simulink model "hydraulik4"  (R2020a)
settings: Solver=ode45  StartTime=0.0  StopTime=2  MaxStep=0.01  RelTol=1e-3  EnableMultiTasking=on
InitFcn:
  | pa = 1e5;

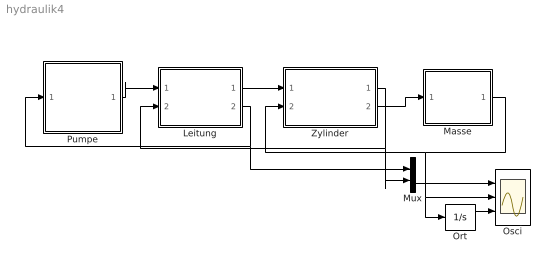
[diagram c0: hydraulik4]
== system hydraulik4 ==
  note: .
  Leitung : Subsystem  mask(Leitung (laminar)){R=8e7}
      mask prompts: R "laminarer Stroemungswiderstand"
  Masse : Subsystem  mask(Masse){m=500}
      mask prompts: m "Masse"
  Mux : Mux  Inputs=2
  Ort : Integrator
  Osci : Scope  NumInputPorts=3
  Pumpe : Subsystem  mask(Pumpe){Qzu=0.001, R=1e9}
      mask prompts: Qzu "Volumenstrom der Pumpe"; R "Stroemungswiderstand der Leckstroemung"
      mask help: Pumpe mit Leckstrom gegen Aussendruck
  Zylinder : Subsystem  mask(Zylinder){A=1e-3, V0=2.5e-5, K=1.15e9, p0=1e5}
      mask prompts: A "Kolbenflaeche"; V0 "Zylindervolumen bei x = 0"; K "Kompressionsmodul"; p0 "Anfangsdruck"
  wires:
  Pumpe/1(Q) -> Leitung/1(Q1)
  Leitung/2(p1) -> Mux/1, Pumpe/1(p)
  Leitung/1(Q2) -> Zylinder/1(Q)
  Zylinder/1(p) -> Mux/2, Leitung/2(p2)
  Zylinder/2(F) -> Masse/1(F)
  Masse/1(v) -> Ort/1, Osci/2, Zylinder/2(v)
  Mux/1 -> Osci/1
  Ort/1 -> Osci/3

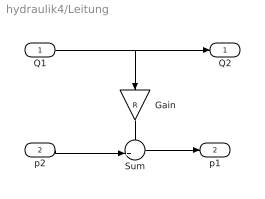
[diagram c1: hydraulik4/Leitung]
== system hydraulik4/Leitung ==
  Q1 : Inport
  p2 : Inport  Port=2
  Gain : Gain  Gain=R
  Sum : Sum  Inputs=++|
  Q2 : Outport
  p1 : Outport  Port=2
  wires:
  Q1/1 -> Q2/1, Gain/1
  p2/1 -> Sum/2
  Sum/1 -> p1/1
  Gain/1 -> Sum/1

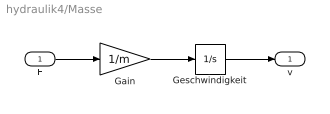
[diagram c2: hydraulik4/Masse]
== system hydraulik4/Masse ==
  F : Inport
  Gain : Gain  Gain=1/m
  Geschwindigkeit : Integrator
  v : Outport
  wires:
  F/1 -> Gain/1
  Geschwindigkeit/1 -> v/1
  Gain/1 -> Geschwindigkeit/1

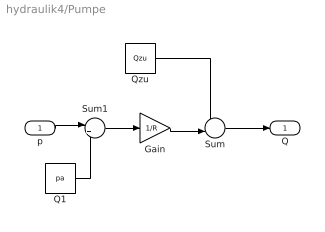
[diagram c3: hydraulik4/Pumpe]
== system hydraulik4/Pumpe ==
  p : Inport
  Gain : Gain  Gain=1/R
  Q1 : Constant  Value=pa
  Qzu : Constant  Value=Qzu
  Sum : Sum  Inputs=+-|
  Sum1 : Sum  Inputs=|+-
  Q : Outport
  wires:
  Qzu/1 -> Sum/1
  Gain/1 -> Sum/2
  Sum/1 -> Q/1
  p/1 -> Sum1/1
  Sum1/1 -> Gain/1
  Q1/1 -> Sum1/2

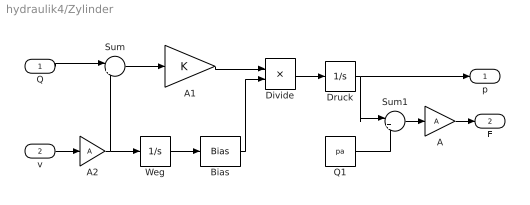
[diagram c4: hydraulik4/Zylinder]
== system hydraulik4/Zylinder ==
  Q : Inport
  v : Inport  Port=2
  A : Gain  Gain=A
  A1 : Gain  Gain=K
  A2 : Gain  Gain=A
  Bias : Bias  Bias=V0
  Divide : Product  Inputs=*/
  Druck : Integrator  InitialCondition=p0  LimitOutput=on  LowerSaturationLimit=0
  Q1 : Constant  Value=pa
  Sum : Sum  Inputs=|+-
  Sum1 : Sum  Inputs=|+-
  Weg : Integrator
  p : Outport
  F : Outport  Port=2
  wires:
  A/1 -> F/1
  Druck/1 -> p/1, Sum1/1
  v/1 -> A2/1
  Weg/1 -> Bias/1
  A2/1 -> Weg/1, Sum/2
  Q/1 -> Sum/1
  Sum/1 -> A1/1
  A1/1 -> Divide/1
  Bias/1 -> Divide/2
  Divide/1 -> Druck/1
  Sum1/1 -> A/1
  Q1/1 -> Sum1/2
